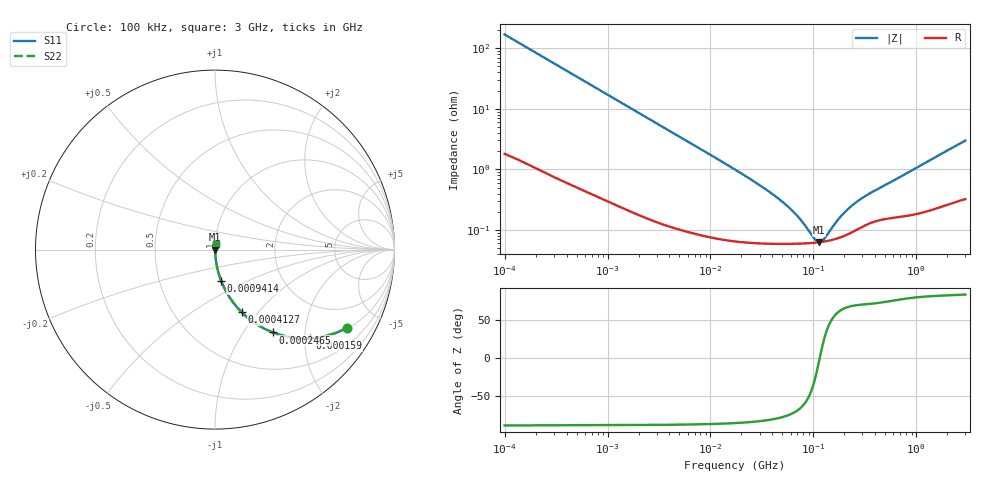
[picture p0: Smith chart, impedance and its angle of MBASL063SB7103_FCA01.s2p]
! MBASL063SB7103_FCA01  S-PARAMETER MODEL  ( Standard Model )
! Model Generated by TAIYO YUDEN Corporation (http://www.ty-top.com)
! Version 1.0
! TAIYO YUDEN Control No. 220601
! Copyright(c) 2020 TAIYO YUDEN CO.,LTD. All Rights Reserved.
! Product Description (link to TY-COMPAS)
! https://ds.yuden.co.jp/TYCOMPAS/or/detail?pn=MBASL063SB7103KFCA01&u=M
! Products Name : Multilayer Ceramic Capacitors
! Characteristics :
!  Capacitance : 0.01 [uF] , Rated Voltage : 10 [V] , TCC : X7R
!  Case Size : 0.6 x 0.3 / 0.024 x 0.012 [mm/inch] , Thickness : 0.3 / 0.012 [mm/inch]
!  (Conditions: Temperature = 25 [degC] , DC Bias Voltage = 0 [V])
! External Node Assignments :
!  1  o---| |---o  2
! GND o---------o GND
! Frequency Range : 100kHz  -  3GHz  [ 401 STEP ]
# MHZ S RI R 50
! Freq[MHz].  S11 Real  S11 Imag  S21 Real  S21 Imag  S12 Real  S12 Imag  S22 Real  S22 Imag
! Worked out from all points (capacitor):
!   401 points, 100 kHz to 3 GHz, reference 50 ohm
!   read as one part in series: C = 9.44 nF near 105.3 kHz
!   lowest |Z| = 63.1 mohm at 113.7 MHz (marker M1)
!   series resonance near 115.4 MHz, so ESL is about 200 pH
!   S11 on the Smith chart (normalised r, x): 100 kHz: 1.04, -3.36; 159 kHz: 1.03, -2.12; 246.5 kHz: 1.02, -1.37; 412.7 kHz: 1.01, -0.82; 941.4 kHz: 1.01, -0.36; 3 GHz: 1.01, +0.06
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0.1  0.7367 -0.4351  0.2633 0.4351  0.2633 0.4351  0.7367 -0.4351
0.159027  0.5296 -0.4932  0.4704 0.4932  0.4704 0.4932  0.5296 -0.4932
0.246461  0.3231 -0.4613  0.6769 0.4613  0.6769 0.4613  0.3231 -0.4613
0.318916  0.2239 -0.4102  0.7761 0.4102  0.7761 0.4102  0.2239 -0.4102
0.412671  0.1488 -0.3489  0.8512 0.3489  0.8512 0.3489  0.1488 -0.3489
0.562235  0.0878 -0.2755  0.9122 0.2755  0.9122 0.2755  0.0878 -0.2755
0.941399  0.0349 -0.1752  0.9651 0.1752  0.9651 0.1752  0.0349 -0.1752
1.659646  0.0126 -0.1023  0.9874 0.1023  0.9874 0.1023  0.0126 -0.1023
3.161081  0.00429 -0.0545  0.9957 0.0545  0.9957 0.0545  0.00429 -0.0545
17.7727  0.000737 -0.00965  0.9993 0.00965  0.9993 0.00965  0.000737 -0.00965
33.85116  0.000619 -0.00475  0.9994 0.00475  0.9994 0.00475  0.000619 -0.00475
52.46276  0.000597 -0.00267  0.9994 0.00267  0.9994 0.00267  0.000597 -0.00267
73.34282  0.000598 -0.00143  0.9994 0.00143  0.9994 0.00143  0.000598 -0.00143
97.38194  0.000613 -0.000522  0.9994 0.000522  0.9994 0.000522  0.000613 -0.000522
105.21  0.00062 -0.000282  0.9994 0.000282  0.9994 0.000282  0.00062 -0.000282
113.6672  0.000629 -4.5e-05  0.9994 4.5e-05  0.9994 4.5e-05  0.000629 -4.5e-05
126.0104  0.000645 0.000272  0.9994 -0.000272  0.9994 -0.000272  0.000645 0.000272
176.1623  0.00074 0.00133  0.9993 -0.00133  0.9993 -0.00133  0.00074 0.00133
240.0085  0.000933 0.0024  0.9991 -0.0024  0.9991 -0.0024  0.000933 0.0024
326.9943  0.00123 0.00351  0.9988 -0.00351  0.9988 -0.00351  0.00123 0.00351
547.5153  0.00159 0.00578  0.9984 -0.00578  0.9984 -0.00578  0.00159 0.00578
3000  0.00411 0.0295  0.9959 -0.0295  0.9959 -0.0295  0.00411 0.0295
